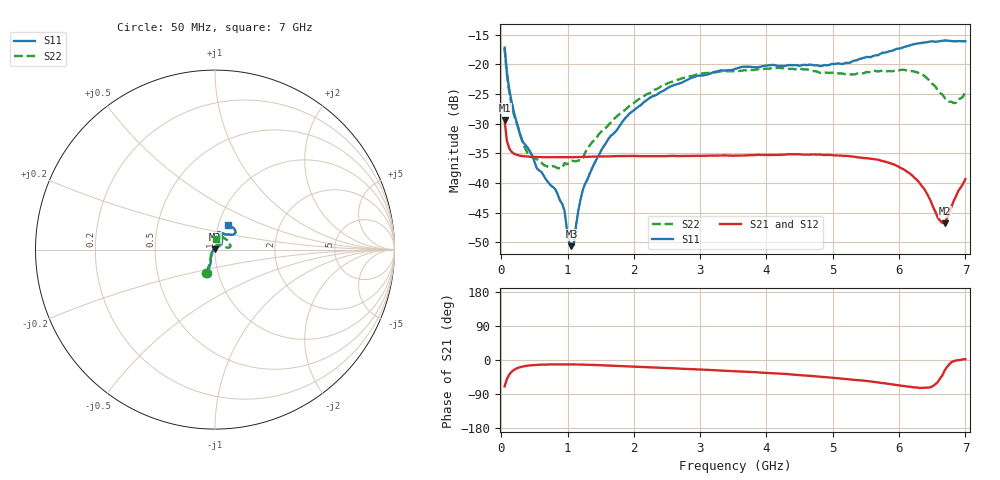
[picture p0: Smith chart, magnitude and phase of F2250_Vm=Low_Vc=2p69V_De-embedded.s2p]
! Integrated Device Technology
! Corporate Headquarters
! 6024 Silver Creek Valley Road
! San Jose, CA 95138  USA
! Phone:  1-408-284-8200
! Toll Free:  1-800-223-1366
! Webpage:  http://www.idt.com/
! Timing and RF Division
! 515 Groton Road, Suite 102
! Westford, MA 01886-6024
! Device:  F2250
! Description: Voltage Variable RF Attenuator
! Frequency:  50.0 -  6000.00 MHz
! Package:  3x3 mm Thin QFN Plastic Package: 16 pin
! Ports:  2 RF, 3 DC
!  Pin  1  = GND
!  Pin  2  = NC
!  Pin  3  = RF1  = Port 1
!  Pin  4  = NC
!  Pin  5  = GND
!  Pin  6  = GND
!  Pin  7  = GND
!  Pin  8  = GND
!  Pin  9  = NC
!  Pin 10  = RF2  = Port 2
!  Pin 11  = NC
!  Pin 12  = GND
!  Pin 13  = GND
!  Pin 14  = VCNTRL
!  Pin 15  = VDD
!  Pin 16  = VMODE
! Vcntrl:  2.690 Volts
! Vmode:  +0.000 Volts
! Vdd:  +3.30  Volts
! Current:  1.176 mA
! Data:  The device was measured on a the F2250 evaluation board which has
!  individual transmission lines to the RF pins.  Data was collected
!  using a calibrated network analyzer.  The evaluation board was
!  de-embedded using a TRL calibration technique.
!  The reference plane is the edge of the package pin.
! Misc:  SN 10
!  Action Tracker AT0258
! Date Measured:  2014-11-26
! Date:  2015-10-15  MJV
! Note:
!  Integrated Device Technology supplies this data as a sample of measured
!  data at the package pin for this product.  Your particular data for this
!  product may vary.
!  Data was taken at 25 degrees C.
!  Integrated Device Technology reserves the right to change this data at anytime.
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# GHz S dB R 50
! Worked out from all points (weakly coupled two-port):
!   201 points, 50 MHz to 7 GHz, reference 50 ohm
!   highest |S21| = -29.41 dB at 50 MHz (marker M1); lowest = -46.8 dB at 6.687 GHz (marker M2)
!   lowest |S11| = -50.7 dB at 1.058 GHz (marker M3), VSWR 1.01, Z = 49.8 + j0.245 ohm
!   |S11| at or under -10 dB: start of sweep to end of sweep
!   |S22| runs from -37.5 to -17.3 dB; largest |S21 - S12| = 5.6e-05
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0.05  -17.18 -108.6  -29.41 -69.8  -29.41 -69.8  -17.28 -111.0
0.08475  -21.45 -107.4  -32.92 -50.3  -32.92 -50.3  -21.74 -110.2
0.15425  -26.23 -116.6  -34.75 -31.1  -34.76 -31.1  -26.81 -122.4
0.29325  -32.21 -127.8  -35.43 -18.5  -35.43 -18.4  -32.10 -137.4
0.3975  -34.08 -141.7  -35.56 -15.0  -35.56 -15.0  -35.04 -160.5
0.5365  -37.56 -155.7  -35.64 -12.8  -35.63 -12.8  -36.04 178.0
0.91875  -43.53 157.9  -35.69 -11.5  -35.68 -11.5  -37.52 133.5
0.9535  -44.68 170.3  -35.69 -11.5  -35.68 -11.5  -36.65 131.0
1.023  -49.95 144.0  -35.67 -11.6  -35.67 -11.6  -36.66 116.0
1.05775  -50.66 122.8  -35.67 -11.6  -35.67 -11.6  -36.28 110.7
1.0925  -50.47 90.0  -35.65 -11.7  -35.66 -11.7  -36.30 106.3
1.162  -44.67 57.0  -35.64 -11.9  -35.64 -11.9  -36.21 95.6
1.2315  -41.09 44.0  -35.61 -12.1  -35.61 -12.1  -35.79 85.9
1.6485  -32.10 42.0  -35.52 -14.6  -35.52 -14.6  -29.88 64.6
2.37825  -24.87 47.3  -35.48 -20.3  -35.48 -20.3  -23.99 56.8
3.525  -20.80 72.5  -35.41 -29.5  -35.41 -29.5  -21.19 74.8
4.7065  -20.17 72.3  -35.21 -42.5  -35.20 -42.5  -21.14 72.3
5.85325  -17.81 40.5  -36.64 -63.3  -36.64 -63.3  -21.13 23.0
6.27025  -16.50 40.1  -39.50 -72.6  -39.51 -72.7  -21.36 9.7
6.68725  -15.99 48.8  -46.84 -27.7  -46.83 -27.4  -25.64 28.5
6.861  -16.13 55.1  -42.18 -1.3  -42.13 -1.3  -26.46 58.0
7  -16.13 63.2  -39.34 1.9  -39.31 1.7  -24.63 83.1
